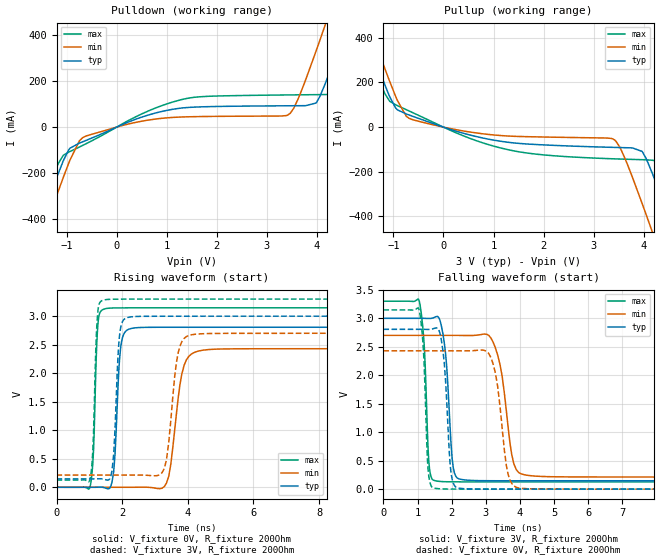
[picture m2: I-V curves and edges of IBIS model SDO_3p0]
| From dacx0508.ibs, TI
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|   Model
[Model]   SDO_3p0
Model_type   Output
Polarity   Non-Inverting
Vmeas = 1.5
Vref = 0
Cref = 1pF
Rref = 100000
|   typ   min   max
C_comp   2.21642pF   1.79332pF   2.6648pF
| Where nom  PVT is Nominal Process, 3.0V, 27C
|   Fast PVT is Strong Process,  3.3V, -40C
|   Slow PVT is Weak Process,   2.7V, 125C
[Voltage Range]   3   2.7   3.3
|Junction Temperature
[Temperature Range]   27   125   -40
[Pullup Reference]   3   2.7   3.3
[Pulldown Reference]   0   0   0
[Power Clamp Reference]   3   2.7   3.3
[GND Clamp Reference]   0   0   0
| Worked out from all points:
|   slope of the pulldown table from 0 to 0.45 V, typ, clamps not added: 11.3 ohm
|   slope of the pullup table from 0 to 0.45 V, typ, clamps not added: 14.7 ohm
|   falling waveform, V_fixture 3V, R_fixture 200Ohm: 20-80 % time 179ps typ, 323ps min, 126ps max; typ from 3 V to 0.147 V
|   rising waveform, V_fixture 0V, R_fixture 200Ohm: 20-80 % time 141ps typ, 306ps min, 101ps max; typ from 0 V to 2.81 V
|   rising waveform, V_fixture 3V, R_fixture 200Ohm: 20-80 % time 133ps typ, 256ps min, 99.8ps max; typ from 0.147 V to 3 V
|   falling waveform, V_fixture 0V, R_fixture 200Ohm: 20-80 % time 162ps typ, 279ps min, 119ps max; typ from 2.81 V to 0 V
[Pulldown]
|   Voltage   I(typ)   I(min)   I(max)
-3V       -1.383A    -1.461A    -1.334A
-1.74V    -560.3mA   -640.6mA   -509.8mA
-1.29V    -276.3mA   -355.7mA   -227.6mA
-1.065V   -146.5mA   -219.1mA   -122.6mA
-606mV    -57.46mA   -38.41mA   -71.8mA
1.329V    83.93mA    44.43mA    121.6mA
3.417V    93.05mA    52.27mA    140.3mA
3.984V    105.1mA    331.4mA    141.5mA
4.173V    192.7mA    449.4mA    142mA
4.65V     486.8mA    754.4mA    254mA
4.902V    648.8mA    917.7mA    410mA
6V        1.366A     1.636A     1.124A
[Pullup]
|   Voltage   I(typ)   I(min)   I(max)
-3V       1.366A     1.439A     1.322A
-1.749V   549.7mA    625mA      503mA
-1.074V   136mA      204.5mA    115.8mA
-615mV    48.56mA    33.25mA    64.91mA
1.275V    -67.36mA   -39.59mA   -100.3mA
3.381V    -90.56mA   -52.6mA    -141.7mA
3.966V    -108.5mA   -340.8mA   -145.8mA
4.173V    -207.5mA   -470.3mA   -148.4mA
4.506V    -411.3mA   -683mA     -188.9mA
4.767V    -577.9mA   -851.6mA   -338.2mA
4.893V    -659.2mA   -933.3mA   -417.3mA
6V        -1.383A    -1.658A    -1.137A
[Ramp]
R_load = 200
|   typ   min   max
dV/dt_r   1.68391/1.41258e-10   1.45763/3.05913e-10   1.88848/1.00573e-10
dV/dt_f   1.71187/1.78517e-10   1.49191/3.23449e-10   1.90378/1.2617e-10
[Falling Waveform]
V_fixture = 3V
V_fixture_min = 2.7V
V_fixture_max = 3.3V
R_fixture = 200Ohm
C_fixture = 0F
|   Time   V(typ)   V(min)   V(max)
0s        3V         2.7V       3.3V
1.05ns    3V         2.7V       3.307V
1.192ns   2.999V     2.7V       2.559V
1.328ns   2.997V     2.7V       501.8mV
1.526ns   3.025V     2.7V       147.3mV
2.046ns   381.1mV    2.7V       129.5mV
2.257ns   174.5mV    2.699V     128.4mV
3.213ns   148mV      2.583V     127.7mV
4.12ns    147.6mV    254.1mV    127.6mV
20ns      146.9mV    213.5mV    127mV
[Rising Waveform]
V_fixture = 0V
V_fixture_min = 0V
V_fixture_max = 0V
R_fixture = 200Ohm
C_fixture = 0F
|   Time   V(typ)   V(min)   V(max)
0s        14.5uV     22.32uV    10.14uV
1.025ns   -63.32uV   -17.54uV   13.71mV
1.266ns   1.454mV    -26.94uV   2.893V
1.461ns   -8.28mV    -34.49uV   3.127V
1.985ns   2.561V     -54.88uV   3.145V
2.257ns   2.781V     -65.46uV   3.146V
3.347ns   2.806V     68.51mV    3.147V
3.82ns    2.806V     1.988V     3.147V
4.316ns   2.806V     2.387V     3.147V
20ns      2.807V     2.429V     3.147V
[Rising Waveform]
V_fixture = 3V
V_fixture_min = 2.7V
V_fixture_max = 3.3V
R_fixture = 200Ohm
C_fixture = 0F
|   Time   V(typ)   V(min)   V(max)
0s        146.9mV    213.5mV    127mV
1.025ns   146.8mV    213.7mV    148.3mV
1.246ns   147.8mV    213.8mV    2.993V
1.423ns   142.8mV    213.8mV    3.28V
1.69ns    290.3mV    213.9mV    3.297V
1.904ns   2.562V     213.9mV    3.298V
2.156ns   2.975V     214mV      3.299V
3.28ns    2.999V     323.3mV    3.299V
4.12ns    3V         2.675V     3.299V
20ns      3V         2.7V       3.3V
[Falling Waveform]
|Gnd
V_fixture = 0V
V_fixture_min = 0V
V_fixture_max = 0V
R_fixture = 200Ohm
C_fixture = 0F
|   Time   V(typ)   V(min)   V(max)
0s        2.807V     2.429V     3.147V
1.05ns    2.807V     2.429V     3.144V
1.308ns   2.805V     2.429V     355mV
1.461ns   2.818V     2.429V     22.2mV
1.742ns   2.442V     2.429V     4.153mV
1.957ns   423.2mV    2.429V     1.894mV
2.156ns   23.51mV    2.429V     1.304mV
3.15ns    878.1uV    2.309V     607uV
3.96ns    836.6uV    20.08mV    578.3uV
20ns      14.51uV    22.62uV    10.45uV
